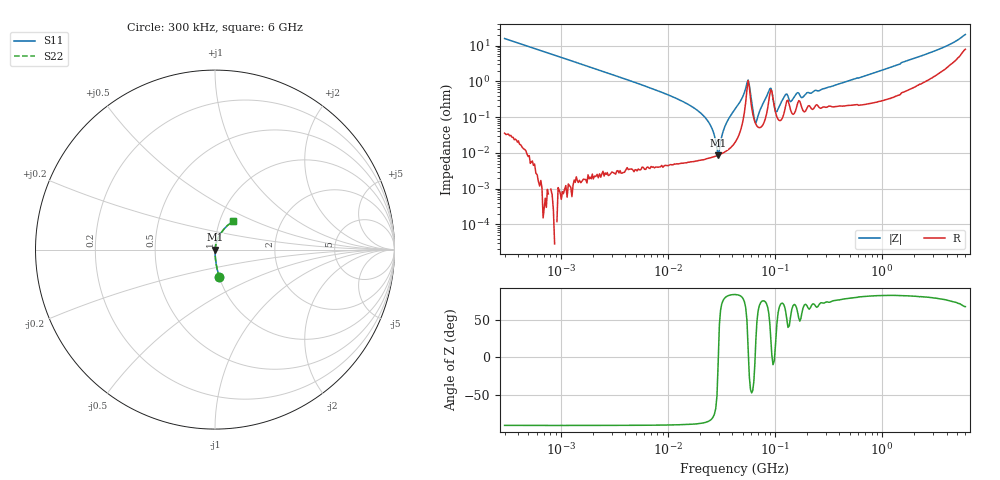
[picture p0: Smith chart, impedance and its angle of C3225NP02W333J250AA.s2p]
! S-Parameter Data Generated by TDK Corporation
! Copyright(C) 2024 TDK Corporation.
! All Rights Reserved.
! TDK P/N: C3225NP02W333J250AA (Multilayer Ceramic Chip Capacitor)
! Property: C=33nF
! Size(LxWxT): 3.2x2.5x2.5mm
! Model Type: s2p (Touchstone File Format Version 1.0)
! Frequency: DC=Yes Start=0.3MHz Stop=6000MHz 402points Log-sweep
! Model Generated on May 28, 2024
! Terms and conditions regarding TDK Simulation Models:
! 1)This simulation model is being provided solely for informational
!  purposes. Please refer to the specifications of the products in
!  terms of detailed characteristics of such products.
! 2)In no event shall TDK Corporation of any of its subsidiaries be
!  liable for any loss or damage arising, directly or indirectly,
!  from any information contained in this simulation model, including,
!  but not limited to loss or damages arising from any inaccuracies,
!  omissions or errors in connection with such information.
! 3)Any and all copyrights on this simulation model are owned by
!  TDK Corporation.  Duplication or redistribution of this simulation
!  model without prior written permission from TDK Corporation
!  is prohibited.
! 4)This simulation model is subject to any modification or change
!  without any prior notice.
! 5)Neither TDK Corporation nor any of its subsidiaries shall make any
!  warranty, express or implied, including but not limited to the
!  correctness, implied warranties of merchantability and fitness for
!  a particular purpose with respect to this simulation models.
! 6)The use of this simulation model shall be deemed to have consented
!  to the terms and conditions hereof.
! Port Assignments:
!  1 ---| |--- 2
! Applicable Conditions:
!  Temperature = 25 degC
!  DC Bias Voltage = 0 V
!  Small Signal Operation
# Hz S MA R 50
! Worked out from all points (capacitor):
!   401 points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, 300 kHz to 6 GHz, reference 50 ohm
!   read as one part in series: C = 33.4 nF near 317.3 kHz
!   lowest |Z| = 8.64 mohm at 29.56 MHz (marker M1)
!   series resonance near 29.64 MHz, so ESL is about 860 pH
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300000  0.1566 -80.9  0.9873 9.0  0.9873 9.0  0.1566 -80.9
1586297  0.02991 -88.3  0.9995 1.7  0.9995 1.7  0.02991 -88.3
8158352  0.00542 -89.3  0.9999 0.3  0.9999 0.3  0.00542 -89.3
2.087273e7  0.001208 -86.9  0.9999 0.1  0.9999 0.1  0.001208 -86.9
2.474969e7  0.0006305 -83.4  0.9999 0.0  0.9999 0.0  0.0006305 -83.4
2.956217e7  8.641e-05 -6.5  0.9999 0.0  0.9999 0.0  8.641e-05 -6.5
3.109046e7  0.0001978 62.2  0.9999 -0.0  0.9999 -0.0  0.0001978 62.2
3.567535e7  0.0007355 80.9  0.9999 -0.0  0.9999 -0.0  0.0007355 80.9
4.28954e7  0.001749 83.2  0.9998 -0.1  0.9998 -0.1  0.001749 83.2
5.481881e7  0.00885 49.1  0.9942 -0.4  0.9942 -0.4  0.00885 49.1
5.772802e7  0.007764 -25.2  0.993 0.2  0.993 0.2  0.007764 -25.2
6.354642e7  0.001099 -32.5  0.9991 0.0  0.9991 0.0  0.001099 -32.5
6.645562e7  0.0006912 23.6  0.9994 -0.0  0.9994 -0.0  0.0006912 23.6
8.968167e7  0.006213 44.5  0.9956 -0.3  0.9956 -0.3  0.006213 44.5
1.04351e8  0.00143 44.3  0.999 -0.1  0.999 -0.1  0.00143 44.3
1.265024e8  0.004348 59.5  0.9978 -0.2  0.9978 -0.2  0.004348 59.5
1.439727e8  0.002929 63.9  0.9987 -0.2  0.9987 -0.2  0.002929 63.9
1.592538e8  0.004583 65.5  0.9981 -0.2  0.9981 -0.2  0.004583 65.5
1.783551e8  0.003494 58.0  0.9982 -0.2  0.9982 -0.2  0.003494 58.0
2.249926e8  0.005007 70.5  0.9983 -0.3  0.9983 -0.3  0.005007 70.5
1.174439e9  0.02422 80.8  0.9964 -1.4  0.9964 -1.4  0.02422 80.8
6e9  0.188 57.3  0.9123 -10.0  0.9123 -10.0  0.188 57.3
